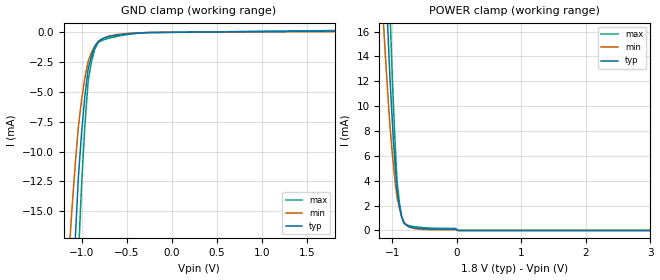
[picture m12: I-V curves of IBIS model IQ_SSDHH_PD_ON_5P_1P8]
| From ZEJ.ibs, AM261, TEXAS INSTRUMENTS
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[Model]   IQ_SSDHH_PD_ON_5P_1P8
Model_type   Input
Polarity   Non-Inverting
Vinl =  0.63
Vinh =  1.17
C_comp   1.313442p   1.241204p   1.780255p
|[Input load] weak_pd_on
|[supplytol] 5
|[temp] ind
[Model Spec]
Vinl   0.63   0.5985   0.6615
Vinh   1.17   1.1115   1.2285
[Temperature Range]   25   125   -40
[Voltage Range]   1.8   1.71   1.89
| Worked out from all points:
|   GND clamp passes 1 mA (typ) near -0.84 V on its own axis
|   POWER clamp passes 1 mA (typ) near -0.85 V on its own axis
| Nom Voltages:
|   VDD=1.1, VDDS=1.8, VDDS18=1.8, BUS_VSSS=0, ESD_BIASFET=0, VSS=0
| Min Voltages:
|   VDD=1.045, VDDS=1.71, VDDS18=1.71, BUS_VSSS=0, ESD_BIASFET=0, VSS=0
| Max Voltages:
|   VDD=1.16, VDDS=1.89, VDDS18=1.89, BUS_VSSS=0, ESD_BIASFET=0, VSS=0
[POWER_clamp]
|   voltage   I(typ)   I(min)   I(max)
-1.8V     125.7mA    90.97mA    174.4mA
-1.145V   25.72mA    17.46mA    37.04mA
-1.109V   21.03mA    14.25mA    30.33mA
-1.073V   16.56mA    11.25mA    23.87mA
-1.036V   12.33mA    8.449mA    17.68mA
-1V       8.805mA    6.198mA    12.37mA
-963.6mV  5.801mA    4.285mA    7.832mA
-927.3mV  3.317mA    2.708mA    4.059mA
-854.5mV  1.094mA    1.108mA    1.113mA
-745.5mV  311.3uA    312.9uA    395.3uA
18.18mV   0A         0A         0A
3.6V      0A         0A         0A
[GND_clamp]
|   voltage   I(typ)   I(min)   I(max)
-1.8V     -190.2mA   -126mA     -287.6mA
-1.145V   -30.72mA   -19.26mA   -48.25mA
-1.109V   -23.91mA   -15.06mA   -37.51mA
-1.073V   -17.75mA   -11.3mA    -27.76mA
-1.036V   -12.25mA   -7.962mA   -18.99mA
-1V       -8.398mA   -5.649mA   -12.78mA
-963.6mV  -5.338mA   -3.804mA   -7.807mA
-927.3mV  -3.068mA   -2.426mA   -4.067mA
-854.5mV  -1.224mA   -1.16mA    -1.399mA
-781.8mV  -588.9uA   -602.5uA   -714.2uA
-272.7mV  -23.46uA   -23.19uA   -31.73uA
1.8V      101.9uA    58.87uA    150.8uA
